(* Logix 5000 AddOnInstructionDefinition export AMCI_SD4840E2_Run_Blend_Move; software revision 20.03 *)

ADD_ON_INSTRUCTION AMCI_SD4840E2_Run_Blend_Move   (* revision 1.0, vendor AMCI, ExecuteEnableInFalse *)
VAR_INPUT
   Axis_Status_Bits : INT; {required}
   Type_0_for_standard_1_for_indexed : BOOL;
   Direction_0_for_CW_1_for_CCW : BOOL; {required}
END_VAR
VAR_IN_OUT
   AMCI_SD4840E2_output_data : _000A:SD4840E2_4342D302:O:0; {required}
END_VAR
VAR_OUTPUT
   EN : BOOL; {access Read Only, visible}
   ER : BOOL; {access Read Only, visible}
END_VAR
VAR
   command_data_block : INT[10];
        [0]   // Command Bits MSW
        [1]   // Command Bits LSW
        [2]   // Upper Target Position
        [3]   // Lower Target Position
        [4]   // Upper Programmed Speed
        [5]   // Lower Programmed Speed
END_VAR

ROUTINE EnableInFalse   (* ladder *)
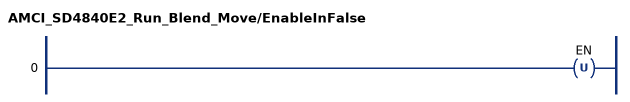
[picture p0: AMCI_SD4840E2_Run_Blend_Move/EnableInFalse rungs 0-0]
   0: OTU(EN);
END_ROUTINE

ROUTINE Logic   (* ladder *)
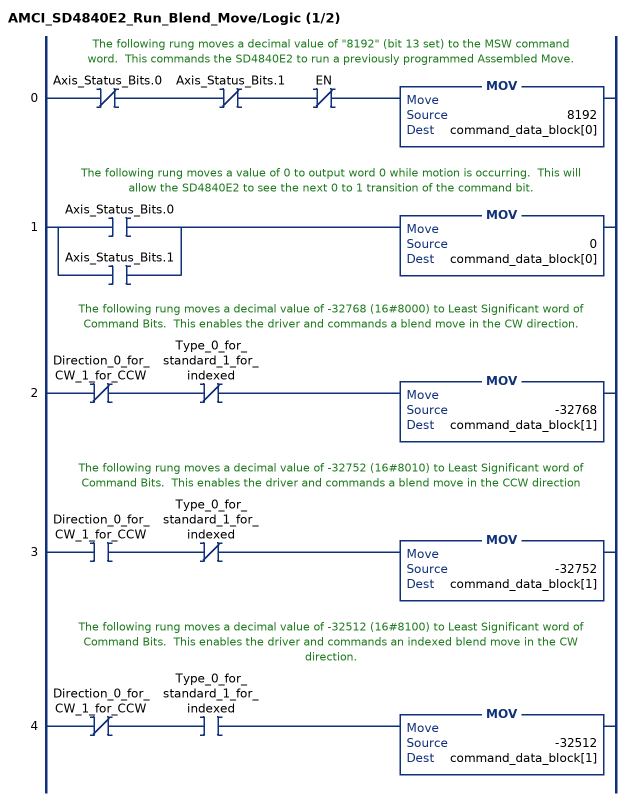
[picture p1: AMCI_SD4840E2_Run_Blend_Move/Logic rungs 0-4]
   // The following rung moves a decimal value of "8192" (bit 13 set) to the MSW command word.  This commands the SD4840E2 to run a previously programmed Assembled Move.
   0: XIO(Axis_Status_Bits.0)XIO(Axis_Status_Bits.1)XIO(EN)MOV(8192,command_data_block[0]);
   // The following rung moves a value of 0 to output word 0 while motion is occurring.  This will allow the SD4840E2 to see the next 0 to 1 transition of the command bit.
   1: [XIC(Axis_Status_Bits.0) ,XIC(Axis_Status_Bits.1) ]MOV(0,command_data_block[0]);
   // The following rung moves a decimal value of -32768 (16#8000) to Least Significant word of Command Bits.  This enables the driver and commands a blend move in the CW direction.
   2: XIO(Direction_0_for_CW_1_for_CCW)XIO(Type_0_for_standard_1_for_indexed)MOV(-32768,command_data_block[1]);
   // The following rung moves a decimal value of -32752 (16#8010) to Least Significant word of Command Bits.  This enables the driver and commands a blend move in the CCW direction
   3: XIC(Direction_0_for_CW_1_for_CCW)XIO(Type_0_for_standard_1_for_indexed)MOV(-32752,command_data_block[1]);
   // The following rung moves a decimal value of -32512 (16#8100) to Least Significant word of Command Bits.  This enables the driver and commands an indexed blend move in the CW direction.
   4: XIO(Direction_0_for_CW_1_for_CCW)XIC(Type_0_for_standard_1_for_indexed)MOV(-32512,command_data_block[1]);
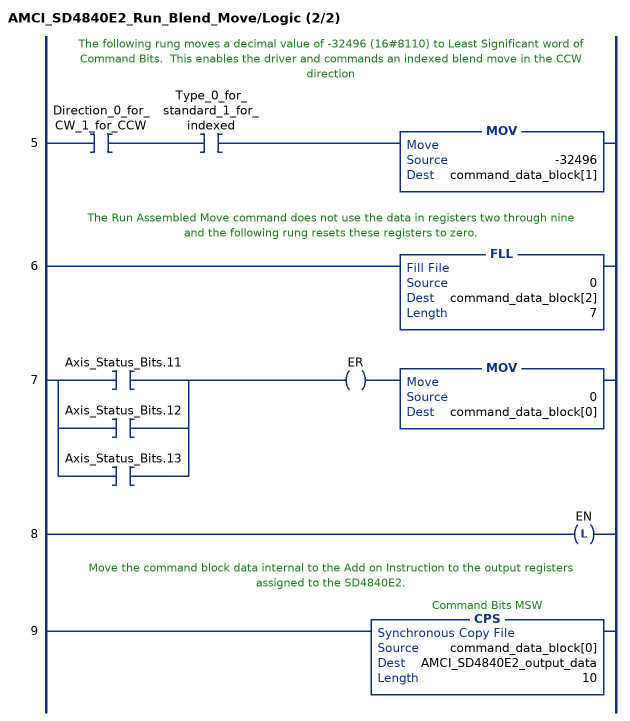
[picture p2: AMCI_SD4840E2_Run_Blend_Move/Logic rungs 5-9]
   // The following rung moves a decimal value of -32496 (16#8110) to Least Significant word of Command Bits.  This enables the driver and commands an indexed blend move in the CCW direction
   5: XIC(Direction_0_for_CW_1_for_CCW)XIC(Type_0_for_standard_1_for_indexed)MOV(-32496,command_data_block[1]);
   // The Run Assembled Move command does not use the data in registers two through nine and the following rung resets these registers to zero.
   6: FLL(0,command_data_block[2],7);
   7: [XIC(Axis_Status_Bits.11) ,XIC(Axis_Status_Bits.12) ,XIC(Axis_Status_Bits.13) ]OTE(ER)MOV(0,command_data_block[0]);
   8: OTL(EN);
   // Move the command block data internal to the Add on Instruction to the output registers assigned to the SD4840E2.
   9: CPS(command_data_block[0],AMCI_SD4840E2_output_data,10);
END_ROUTINE
END_ADD_ON_INSTRUCTION
